// Crossing with 4 TrafficLights
(*
			|		|
		  TL|		|
		  V2|		|TLH2
------------ --	 	 -------------
					|			
			|
------------	  -- -------------
		TLH1|		|TL
			|		|V1
			|		|
*)
FUNCTION_BLOCK FB_Crossing
VAR_INPUT
	// name
	sInName						: STRING; 	// name of crossing
	
	// commissioning mode
	bInCommissioning			: BOOL; 	// sensor signal commissioning mode (on rising edge)
	
	// automatic mode
	bInAutomatic				: BOOL; 	// sensor signal automatic mode (on rising edge)
	
	// automatic Active
	bInAutomaticActive			: BOOL; 	// sensor signal automatic active mode (on rising edge) -> traffic lights H1/2 and V1/2 alternate 
	
	// automatic stand by
	bInAutomaticStandBy			: BOOL;		// sensor signal automatic stand by mode (on rising edge) -> on all traffic lights the yellow light blinks  
	
END_VAR
VAR_OUTPUT
	// commissioning mode
	bOutCommissioningMode		: BOOL;		// status signal commissioning mode active
	
	// automatic mode
	bOutAutomaticMode			: BOOL;		// status signal automatic mode active

	// traffic lights
	fbTrafficLightH1	: FB_SingleTrafficLight;	// traffic light horizontal 1 (TLH1)
	fbTrafficLightH2	: FB_SingleTrafficLight;	// traffic light horizontal 2 (TLH2)
	fbTrafficLightV1	: FB_SingleTrafficLight;	// traffic light vertical 1 (TLV1)
	fbTrafficLightV2	: FB_SingleTrafficLight;	// traffic light vertical 2 (TLV2)
END_VAR
VAR
	// commissioning mode
	eOpmodeState				: E_CrossOpmodeState;			// opmode state
	fbRTrigInCommissioning		: R_TRIG;						// rising edge detection
	
	// automatic mode
	eAutomaticState				: E_CrossAutomaticState;		// automatic state
	fbRTrigInAutomatic			: R_TRIG;						// rising edge detection
	
	// automatic active
	eAutomaticActiveState		: E_CrossAutomaticActiveState;	// automatic active state
	fbRTrigInAutomaticActive	: R_TRIG;						// rising edge detection
	fbTimerReleaseH				: TON;							// timer horizontal traffic
	fbTimerWaitBeforeV			: TON;							// timer for waiting before releasing vertical traffic 
	fbTimerReleaseV				: TON;							// timer vertical traffic 
	fbTimerWaitBeforeH			: TON;							// timer for waiting before releasing horizontal traffic 
	
	// automatic stand by
	fbRTrigInAutomaticStandBy	: R_TRIG;						// rising edge detection
	
	// HMI data
	stHmiData					:ST_CrossHmiData;				// hmi data to interaction with hmi
	
END_VAR

METHOD FB_init : BOOL
VAR_INPUT
	bInitRetains : BOOL; // if TRUE, the retain variables are initialized (warm start / cold start)
	bInCopyCode : BOOL;  // if TRUE, the instance afterwards gets moved into the copy code (online change)
END_VAR
sInName := 'Crossing';
fbTrafficLightH1.sInName :=  'TL Horizontal 1';
fbTrafficLightH2.sInName :=  'TL Horizontal 2';
fbTrafficLightV1.sInName :=  'TL Vertical 1';
fbTrafficLightV2.sInName :=  'TL Vertical 2';
END_METHOD

METHOD M_AutoActiveHTGreenRequest : BOOL
VAR_INPUT
END_VAR
// horizontal traffic green request
fbTrafficLightH1.bInRedRequest 		:= FALSE;
fbTrafficLightH1.bInGreenRequest 	:= TRUE;
fbTrafficLightH2.bInRedRequest 		:= FALSE;
fbTrafficLightH2.bInGreenRequest 	:= TRUE;
			
fbTrafficLightV1.bInRedRequest 		:= FALSE;
fbTrafficLightV1.bInGreenRequest	:= FALSE;
fbTrafficLightV2.bInRedRequest 		:= FALSE;
fbTrafficLightV2.bInGreenRequest	:= FALSE;
END_METHOD

METHOD M_AutoActiveHTRedRequest : BOOL
VAR_INPUT
END_VAR
// horizontal traffic red request
fbTrafficLightH1.bInRedRequest		:= TRUE;
fbTrafficLightH1.bInGreenRequest 	:= FALSE;
fbTrafficLightH2.bInRedRequest 		:= TRUE;
fbTrafficLightH2.bInGreenRequest 	:= FALSE;
			
fbTrafficLightV1.bInRedRequest 		:= FALSE;
fbTrafficLightV1.bInGreenRequest 	:= FALSE;
fbTrafficLightV2.bInRedRequest 		:= FALSE;
fbTrafficLightV2.bInGreenRequest 	:= FALSE;
END_METHOD

METHOD M_AutoActiveVTGreenRequest : BOOL
VAR_INPUT
END_VAR
// vertical traffic green request
fbTrafficLightV1.bInRedRequest 		:= FALSE;
fbTrafficLightV1.bInGreenRequest 	:= TRUE;
fbTrafficLightV2.bInRedRequest 		:= FALSE;
fbTrafficLightV2.bInGreenRequest 	:= TRUE;
			
fbTrafficLightH1.bInRedRequest 		:= FALSE;
fbTrafficLightH1.bInGreenRequest	:= FALSE;
fbTrafficLightH2.bInRedRequest 		:= FALSE;
fbTrafficLightH2.bInGreenRequest	:= FALSE;
END_METHOD

METHOD M_AutoActiveVTRedRequest : BOOL
VAR_INPUT
END_VAR
// vertical traffic red request
fbTrafficLightV1.bInRedRequest		:= TRUE;
fbTrafficLightV1.bInGreenRequest 	:= FALSE;
fbTrafficLightV2.bInRedRequest 		:= TRUE;
fbTrafficLightV2.bInGreenRequest 	:= FALSE;
			
fbTrafficLightH1.bInRedRequest 		:= FALSE;
fbTrafficLightH1.bInGreenRequest 	:= FALSE;
fbTrafficLightH2.bInRedRequest 		:= FALSE;
fbTrafficLightH2.bInGreenRequest 	:= FALSE;
END_METHOD

METHOD M_Automatic : BOOL
VAR_INPUT
END_VAR
// automatic state machine
CASE eAutomaticState OF

	eCrossAutomatic_StandBy:
		M_AutomaticStandBy();
		IF fbRTrigInAutomaticActive.Q AND NOT fbRTrigInAutomaticStandBy.Q  THEN
			//IF M_SetAutomaticActiveModeTrafficLights() THEN
				eAutomaticActiveState := eCrossAutoActive_WaitBeforeH;
				eAutomaticState := eCrossAutomatic_Active;
			//END_IF
		END_IF

	eCrossAutomatic_Active:
		M_AutomaticActive();
		IF NOT fbRTrigInAutomaticActive.Q  AND fbRTrigInAutomaticStandBy.Q THEN
			//IF M_SetAutomaticStandByModeTrafficLights() THEN
				eAutomaticState := eCrossAutomatic_StandBy;
			//END_IF			
		END_IF
		
END_CASE
END_METHOD

METHOD M_AutomaticActive : BOOL
VAR_INPUT
END_VAR
// automatic active mode state machine
CASE eAutomaticActiveState OF
	
	// horizontal traffic will be released if vertical traffic stops
	eCrossAutoActive_WaitBeforeH:
		fbTimerReleaseH(PT:=T#2S);
		
		IF fbTrafficLightV1.bOutRedRequestReady AND fbTrafficLightV2.bOutRedRequestReady THEN
			fbTimerReleaseH.IN := TRUE;
		END_IF
		
		IF fbTimerReleaseH.Q THEN
			fbTimerReleaseH(IN:=FALSE);
			eAutomaticActiveState := eCrossAutoActive_ReleaseH;
		END_IF
	
	// horizontal traffic is released	
	eCrossAutoActive_ReleaseH:
		fbTimerWaitBeforeV(PT:=T#2S);
		
		IF fbTrafficLightH1.bOutGreenRequestReady AND fbTrafficLightH2.bOutGreenRequestReady THEN
			fbTimerWaitBeforeV.IN := TRUE;
		END_IF	
	
		IF fbTimerWaitBeforeV.Q THEN
			fbTimerWaitBeforeV(IN:=FALSE);
			eAutomaticActiveState := eCrossAutoActive_WaitBeforeV;
		END_IF
	
	// vertical traffic will be released if horizontal traffic stops
	eCrossAutoActive_WaitBeforeV:
		fbTimerReleaseV(PT:=T#2S);
		
		IF fbTrafficLightH1.bOutRedRequestReady AND fbTrafficLightH2.bOutRedRequestReady THEN
			fbTimerReleaseV.IN := TRUE;
		END_IF
		
		IF fbTimerReleaseV.Q THEN
			fbTimerReleaseV(IN:=FALSE);
			eAutomaticActiveState := eCrossAutoActive_ReleaseV;
		END_IF
	
	// vertical traffc is released	
	eCrossAutoActive_ReleaseV:
		fbTimerWaitBeforeH(PT:=T#2S);
		
		IF fbTrafficLightV1.bOutGreenRequestReady AND fbTrafficLightV2.bOutGreenRequestReady THEN
			fbTimerWaitBeforeH.IN := TRUE;
		END_IF	
		
		IF fbTimerWaitBeforeH.Q THEN
			fbTimerWaitBeforeH(IN:=FALSE);
			eAutomaticActiveState := eCrossAutoActive_WaitBeforeH;
		END_IF
	
END_CASE
END_METHOD

METHOD M_AutomaticStandBy : BOOL
VAR_INPUT
END_VAR
// reset timers
fbTimerReleaseH(IN:=FALSE);
fbTimerWaitBeforeV(IN:=FALSE);
fbTimerReleaseV(IN:=FALSE);
fbTimerWaitBeforeH(IN:=FALSE);
// implement additional functions for automatic stand by mode
END_METHOD

METHOD M_Commissioning : BOOL
VAR_INPUT
END_VAR
// implement additional functions for commissioning mode
END_METHOD

METHOD M_Cycle : BOOL
VAR_INPUT
END_VAR
// process input signals
M_Input();

// opmode state machine
CASE eOpmodeState OF
	
	eCrossOpmode_Commissioning:
		M_Commissioning();
		IF fbRTrigInAutomatic.Q AND NOT fbRTrigInCommissioning.Q THEN
			//IF M_SetAutomaticStandByModeTrafficLights() THEN
				eAutomaticState := eCrossAutomatic_StandBy;
				eOpmodeState := eCrossOpmode_Automatic;
			//END_IF
		END_IF
		
	eCrossOpmode_Automatic:
		M_Automatic();
		IF NOT fbRTrigInAutomatic.Q AND fbRTrigInCommissioning.Q THEN
			//IF M_SetCommissioningModeTrafficLights() THEN
				eOpmodeState := eCrossOpmode_Commissioning;
			//END_IF		
		END_IF

END_CASE

// set output signals
M_Output();
END_METHOD

METHOD M_Input : BOOL
VAR_INPUT
END_VAR
// process input signals

// commissioning mode
fbRTrigInCommissioning(CLK := bInCommissioning OR stHmiData.bInCommissioning);

// automatic mode
fbRTrigInAutomatic(CLK := bInAutomatic OR stHmiData.bInAutomatic);

// automatic Active
fbRTrigInAutomaticActive(CLK := bInAutomaticActive OR stHmiData.bInAutomaticActive);

// automatic stand by
fbRTrigInAutomaticStandBy(CLK := bInAutomaticStandBy OR stHmiData.bInAutomaticStandBy);
END_METHOD

METHOD M_Output : BOOL
VAR_INPUT
END_VAR
// set output signals

// execute traffic lights
fbTrafficLightH1.M_Cycle();
fbTrafficLightH2.M_Cycle();
fbTrafficLightV1.M_Cycle();
fbTrafficLightV2.M_Cycle();

IF eOpmodeState = eCrossOpmode_Automatic THEN
	// automatic mode
	bOutCommissioningMode := FALSE;
	bOutAutomaticMode := TRUE;
	M_SetAutomaticModeTrafficLights();
		
	IF eAutomaticState = eCrossAutomatic_Active THEN
		// automatic active mode
		M_SetAutomaticActiveModeTrafficLights();
			
		IF eAutomaticActiveState = eCrossAutoActive_WaitBeforeH THEN
			// vertical traffic red request
			M_AutoActiveVTRedRequest();
			
		ELSIF eAutomaticActiveState = eCrossAutoActive_ReleaseH THEN
			// horizontal traffic green request
			M_AutoActiveHTGreenRequest();
			
		ELSIF eAutomaticActiveState = eCrossAutoActive_WaitBeforeV THEN
			// horizontal traffic red request
			M_AutoActiveHTRedRequest();
			
		ELSIF eAutomaticActiveState = eCrossAutoActive_ReleaseV THEN
			// vertical traffic green request
			M_AutoActiveVTGreenRequest();
		END_IF
		
	ELSIF eAutomaticState = eCrossAutomatic_StandBy THEN
		// automatic stand by mode
		M_SetAutomaticStandByModeTrafficLights();
	ELSE
		// automatic stand by mode
		M_SetAutomaticStandByModeTrafficLights();
					
	END_IF

	
ELSIF eOpmodeState = eCrossOpmode_Commissioning THEN
	// commissioning mode
	bOutCommissioningMode := TRUE;
	bOutAutomaticMode := FALSE;
	M_SetCommissioningModeTrafficLights();
	
ELSE
	// commissioning mode
	bOutCommissioningMode := TRUE;
	bOutAutomaticMode := FALSE;
	M_SetCommissioningModeTrafficLights();
	
END_IF

// hmi output data
stHmiData.sOutName := sInName;
stHmiData.bOutCommissioningMode := bOutCommissioningMode;
stHmiData.bOutAutomaticMode := bOutAutomaticMode;
END_METHOD

METHOD M_SetAutomaticActiveModeTrafficLights : BOOL
VAR_INPUT
END_VAR
// set all traffic lights to automatic active mode
fbTrafficLightH1.bInAutomaticStandBy := FALSE;
fbTrafficLightH2.bInAutomaticStandBy := FALSE;
fbTrafficLightV1.bInAutomaticStandBy := FALSE;
fbTrafficLightV2.bInAutomaticStandBy := FALSE;

fbTrafficLightH1.bInAutomaticActive := TRUE;
fbTrafficLightH2.bInAutomaticActive := TRUE;
fbTrafficLightV1.bInAutomaticActive := TRUE;
fbTrafficLightV2.bInAutomaticActive := TRUE;

fbTrafficLightV1.bInRedRequest 			:= FALSE;
fbTrafficLightV1.bInGreenRequest 		:= FALSE;
fbTrafficLightV2.bInRedRequest 			:= FALSE;
fbTrafficLightV2.bInGreenRequest 		:= FALSE;	

fbTrafficLightH1.bInRedRequest 			:= FALSE;
fbTrafficLightH1.bInGreenRequest 		:= FALSE;
fbTrafficLightH2.bInRedRequest 			:= FALSE;
fbTrafficLightH2.bInGreenRequest 		:= FALSE;

M_SetAutomaticActiveModeTrafficLights := TRUE;
END_METHOD

METHOD M_SetAutomaticModeTrafficLights : BOOL
VAR_INPUT
END_VAR
// set all traffic lights to automatic mode

// vertical traffic automatic mode
fbTrafficLightV1.bInCommissioning 	:= FALSE;
fbTrafficLightV2.bInCommissioning 	:= FALSE;
fbTrafficLightV1.bInAutomatic 		:= TRUE;
fbTrafficLightV2.bInAutomatic 		:= TRUE;
// horizontal traffic automatic mode
fbTrafficLightH1.bInCommissioning 	:= FALSE;
fbTrafficLightH2.bInCommissioning 	:= FALSE;
fbTrafficLightH1.bInAutomatic 		:= TRUE;
fbTrafficLightH2.bInAutomatic 		:= TRUE;

M_SetAutomaticModeTrafficLights := TRUE;
END_METHOD

METHOD M_SetAutomaticStandByModeTrafficLights : BOOL
VAR_INPUT
END_VAR
// set all traffic lights to automatic stand by mode

fbTrafficLightH1.bInAutomaticActive := FALSE;
fbTrafficLightH2.bInAutomaticActive := FALSE;
fbTrafficLightV1.bInAutomaticActive := FALSE;
fbTrafficLightV2.bInAutomaticActive := FALSE;

fbTrafficLightH1.bInAutomaticStandBy := TRUE;
fbTrafficLightH2.bInAutomaticStandBy := TRUE;
fbTrafficLightV1.bInAutomaticStandBy := TRUE;
fbTrafficLightV2.bInAutomaticStandBy := TRUE;

// reset request signals
fbTrafficLightV1.bInRedRequest 			:= FALSE;
fbTrafficLightV1.bInGreenRequest 		:= FALSE;
fbTrafficLightV2.bInRedRequest 			:= FALSE;
fbTrafficLightV2.bInGreenRequest 		:= FALSE;		
	
fbTrafficLightH1.bInRedRequest 			:= FALSE;
fbTrafficLightH1.bInGreenRequest 		:= FALSE;
fbTrafficLightH2.bInRedRequest 			:= FALSE;
fbTrafficLightH2.bInGreenRequest 		:= FALSE;

M_SetAutomaticStandByModeTrafficLights := TRUE;
END_METHOD

METHOD M_SetCommissioningModeTrafficLights : BOOL
VAR_INPUT
END_VAR
// set all traffic lights to commissioning mode

fbTrafficLightH1.bInAutomatic := FALSE;
fbTrafficLightH2.bInAutomatic := FALSE;
fbTrafficLightV1.bInAutomatic := FALSE;
fbTrafficLightV2.bInAutomatic := FALSE;

fbTrafficLightH1.bInAutomaticActive := FALSE;
fbTrafficLightH2.bInAutomaticActive := FALSE;
fbTrafficLightV1.bInAutomaticActive := FALSE;
fbTrafficLightV2.bInAutomaticActive := FALSE;

fbTrafficLightH1.bInAutomaticStandBy := TRUE;
fbTrafficLightH2.bInAutomaticStandBy := TRUE;
fbTrafficLightV1.bInAutomaticStandBy := TRUE;
fbTrafficLightV2.bInAutomaticStandBy := TRUE;

fbTrafficLightH1.bInCommissioning := TRUE;
fbTrafficLightH2.bInCommissioning := TRUE;
fbTrafficLightV1.bInCommissioning := TRUE;
fbTrafficLightV2.bInCommissioning := TRUE;

M_SetCommissioningModeTrafficLights := TRUE;
END_METHOD

END_FUNCTION_BLOCK
